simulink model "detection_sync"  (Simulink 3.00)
settings: Solver=ode113  StartTime=0.0  StopTime=0.1  RelTol=1e-3
undefined symbols (not defined in the file or in its folder): tout

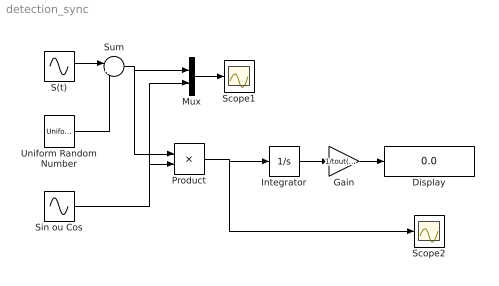
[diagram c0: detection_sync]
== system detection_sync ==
  Display : Display
  Gain : Gain  Gain=1/tout(length(tout))  SaturateOnIntegerOverflow=on
  Integrator : Integrator  ExternalReset=none  InitialConditionSource=internal  InitialCondition=0  LimitOutput=off  UpperSaturationLimit=inf  LowerSaturationLimit=-inf  ShowSaturationPort=off  ShowStatePort=off  AbsoluteTolerance=auto
  Mux : Mux  Description=Mux  Inputs=2
  Product : Product  Inputs=2  SaturateOnIntegerOverflow=on
  S(t) : Sin  Amplitude=1  Frequency=1000  Phase=0  SampleTime=0
  Scope1 : Scope
  Scope2 : Scope
  Sin ou Cos : Sin  Amplitude=1  Frequency=1000  Phase=0  SampleTime=0
  Sum : Sum  Inputs=|++  SaturateOnIntegerOverflow=on
  Uniform Random Number : UniformRandomNumber  Minimum=-1  Maximum=1  Seed=0  SampleTime=0
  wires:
  Integrator/1 -> Gain/1
  Gain/1 -> Display/1
  Mux/1 -> Scope1/1
  Product/1 -> Integrator/1, Scope2/1
  S(t)/1 -> Sum/1
  Uniform Random Number/1 -> Sum/2
  Sum/1 -> Mux/1, Product/1
  Sin ou Cos/1 -> Product/2, Mux/2
